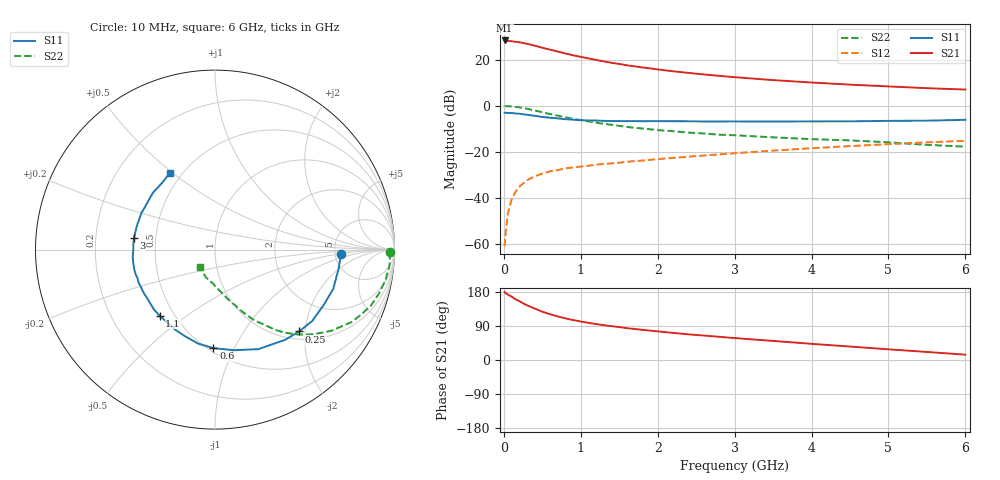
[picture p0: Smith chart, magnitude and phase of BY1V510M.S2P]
! SIEMENS Small Signal Semiconductors
! BFY420
! Si NPN RF SIEGET Grounded Emitter Transistor in MICRO-X
! VCE = 1.5 V  IC = 10 mA
! Common Emitter S-Parameters:  October  1996
# GHz  S  MA  R  50
!  f  S11  S21  S12  S22
! GHz  MAG  ANG  MAG  ANG  MAG  ANG  MAG  ANG
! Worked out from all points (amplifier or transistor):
!   36 points, 10 MHz to 6 GHz, reference 50 ohm
!   highest |S21| = 28.3 dB at 10 MHz (marker M1)
!   |S21| within 3 dB of that: start of sweep to 481.9 MHz
!   unconditionally stable (mu >= 1): 2.453 GHz to end of sweep
!   at 250 MHz: K = 0.19, MSG = 30.5 dB, |S12| = -33.8 dB
!   at 1.4 GHz: K = 0.76, MSG = 21.8 dB, |S12| = -25.0 dB
!   at 6 GHz: K = 1.10, MAG = 9.1 dB, |S12| = -15.2 dB
!   S11 on the Smith chart (normalised r, x): 10 MHz: 5.66, -0.57; 250 MHz: 1.17, -1.86; 600 MHz: 0.53, -0.83; 1.1 GHz: 0.42, -0.40; 3 GHz: 0.37, +0.06; 6 GHz: 0.43, +0.49
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0.01  0.7022 -2.1  26.02 179.4  0.0009 97.4  0.9779 -0.9
0.02  0.7 -4.1  25.85 176.8  0.0015 89.4  0.9751 -1.8
0.05  0.6965 -9.2  25.32 172.9  0.0045 87.3  0.9765 -5.0
0.1  0.6943 -18.5  25.08 167.5  0.0091 79.9  0.9654 -10.1
0.15  0.6795 -27.2  24.36 160.5  0.0134 76.4  0.9454 -15.1
0.2  0.672 -36.3  23.82 155.5  0.0174 74.1  0.924 -19.6
0.25  0.6539 -44.2  22.95 149.6  0.0205 69.2  0.8909 -24.0
0.3  0.6366 -52.2  22 144.5  0.0242 67.2  0.8605 -28.0
0.4  0.6047 -66.5  20.1 135.9  0.0294 61.7  0.7894 -35.0
0.5  0.5707 -79.2  18.07 127.4  0.0337 57.4  0.7224 -40.8
0.6  0.5492 -90.9  16.46 120.9  0.0378 54.6  0.6623 -45.6
0.8  0.5104 -109.2  13.57 109.9  0.0438 49.6  0.561 -53.0
0.9  0.4982 -116.4  12.42 105.4  0.0459 48.7  0.5199 -55.4
1.1  0.4798 -130.0  10.63 98.0  0.0501 48.0  0.4561 -60.5
1.3  0.4692 -139.7  9.142 91.9  0.0548 46.9  0.404 -63.9
1.6  0.4626 -153.2  7.532 84.0  0.0608 46.1  0.3477 -68.7
2.2  0.4613 -171.1  5.577 71.5  0.0739 45.4  0.2803 -76.1
3  0.4566 171.9  4.159 57.9  0.0933 43.1  0.229 -84.0
3.5  0.4549 162.2  3.591 50.3  0.1062 40.6  0.2063 -89.0
4.5  0.4584 145.7  2.865 35.5  0.133 34.0  0.177 -99.5
5.5  0.4746 128.3  2.399 21.2  0.1606 25.9  0.1419 -118.0
6  0.4944 120.8  2.241 14.1  0.1736 21.5  0.1293 -131.2
